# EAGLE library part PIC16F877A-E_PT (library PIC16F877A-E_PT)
8-bit Microcontrollers - MCU 14KB 368 RAM 33 I/O Source: Datasheet
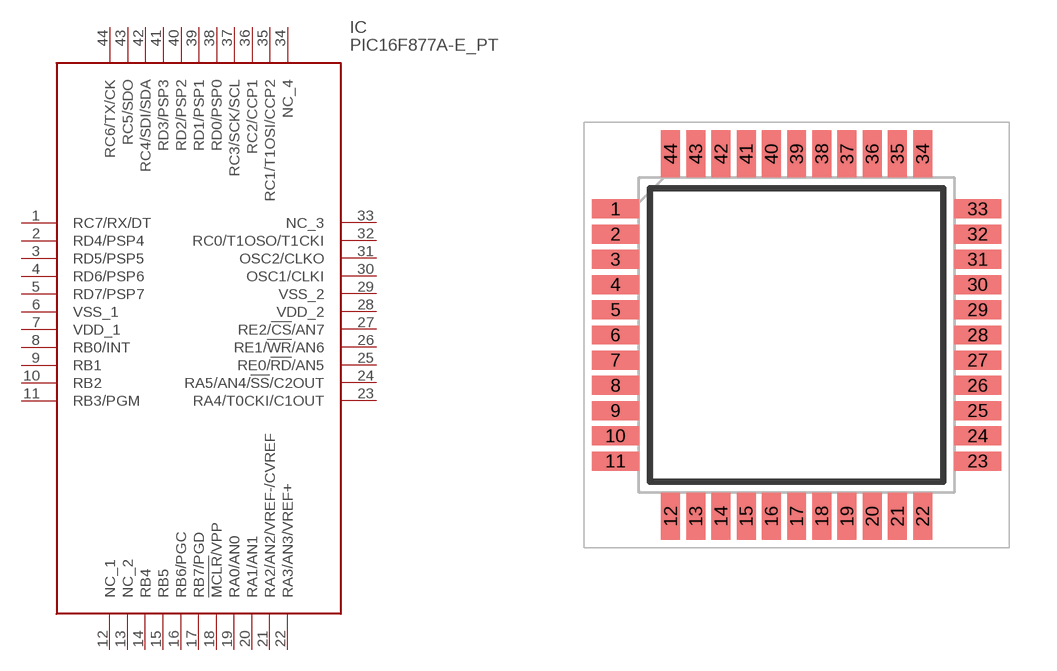
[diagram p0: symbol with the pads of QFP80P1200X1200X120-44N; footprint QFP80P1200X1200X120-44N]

Designator prefix IC

## PIC16F877A-E_PT (Description: 8-bit Microcontrollers - MCU 14KB 368 RAM 33 I/O; Height: 1.2mm; Manufacturer_Name: Microchip; Manufacturer_Part_Number: PIC16F877A-E/PT; Mouser_Part_Number: 579-PIC16F877A-E/PT; Mouser_Price-Stock: https://www.mouser.co.uk/ProductDetail/Microchip-Technology/PIC16F877A-E-PT?qs=rh436G1KrYyphrErQ8h5Pw%3D%3D)  [QFP80P1200X1200X120-44N]
1  RC7/RX/DT
2  RD4/PSP4
3  RD5/PSP5
4  RD6/PSP6
5  RD7/PSP7
6  VSS_1
7  VDD_1
8  RB0/INT
9  RB1
10  RB2
11  RB3/PGM
12  NC_1
13  NC_2
14  RB4
15  RB5
16  RB6/PGC
17  RB7/PGD
18  !MCLR!/VPP
19  RA0/AN0
20  RA1/AN1
21  RA2/AN2/VREF-/CVREF
22  RA3/AN3/VREF+
23  RA4/T0CKI/C1OUT
24  RA5/AN4/!SS!/C2OUT
25  RE0/!RD!/AN5
26  RE1/!WR!/AN6
27  RE2/!CS!/AN7
28  VDD_2
29  VSS_2
30  OSC1/CLKI
31  OSC2/CLKO
32  RC0/T1OSO/T1CKI
33  NC_3
34  NC_4
35  RC1/T1OSI/CCP2
36  RC2/CCP1
37  RC3/SCK/SCL
38  RD0/PSP0
39  RD1/PSP1
40  RD2/PSP2
41  RD3/PSP3
42  RC4/SDI/SDA
43  RC5/SDO
44  RC6/TX/CK

## Footprint QFP80P1200X1200X120-44N (pad centres in mm)
44-Lead Plastic Thin Quad Flatpack (PT) 10x10x1 mm Body, 1.0/0.10 mm L ead Form (TQFP)
smd 1.5 x 0.6: 1 -5.75,4; 2 -5.75,3.2; 3 -5.75,2.4; 4 -5.75,1.6; 5 -5.75,0.8; 6 -5.75,0; 7 -5.75,-0.8; 8 -5.75,-1.6; 9 -5.75,-2.4; 10 -5.75,-3.2; 11 -5.75,-4; 23 5.75,-4; 24 5.75,-3.2; 25 5.75,-2.4; 26 5.75,-1.6; 27 5.75,-0.8; 28 5.75,0; 29 5.75,0.8; 30 5.75,1.6; 31 5.75,2.4; 32 5.75,3.2; 33 5.75,4
smd 0.6 x 1.5: 12 -4,-5.75; 13 -3.2,-5.75; 14 -2.4,-5.75; 15 -1.6,-5.75; 16 -0.8,-5.75; 17 0,-5.75; 18 0.8,-5.75; 19 1.6,-5.75; 20 2.4,-5.75; 21 3.2,-5.75; 22 4,-5.75; 34 4,5.75; 35 3.2,5.75; 36 2.4,5.75; 37 1.6,5.75; 38 0.8,5.75; 39 0,5.75; 40 -0.8,5.75; 41 -1.6,5.75; 42 -2.4,5.75; 43 -3.2,5.75; 44 -4,5.75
